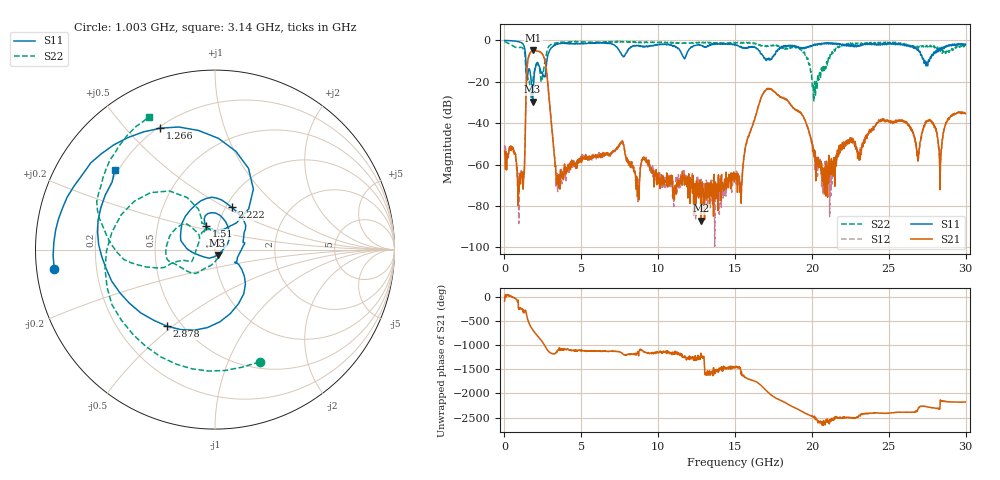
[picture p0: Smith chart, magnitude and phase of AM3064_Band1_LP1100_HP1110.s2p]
# Hz S DB R 50.0
!freq dBS11 angS11 dBS21 angS21 dBS12 angS12 dBS22 angS22
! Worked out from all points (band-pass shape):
!   1600 points, 10 MHz to 29.98 GHz, reference 50 ohm
!   highest |S21| = -4.83 dB at 1.884 GHz (marker M1); lowest = -87.1 dB at 12.77 GHz (marker M2)
!   |S21| within 3 dB of the highest: 1.578 GHz to 2.553 GHz (975.3 MHz wide, 47.2 % of centre)
!   lowest |S11| = -29.7 dB at 1.828 GHz (marker M3), VSWR 1.07, Z = 51.4 - j3.04 ohm
!   |S11| at or under -10 dB: 1.393 GHz to 2.759 GHz (1.366 GHz wide, 65.8 % of centre); 27.28266 GHz to 27.35234 GHz (69.67 MHz wide, 0.255 % of centre); 27.36 GHz to 27.57 GHz (208.9 MHz wide, 0.761 % of centre)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
!   |S22| runs from -29.5 to -0.5 dB; largest |S21 - S12| = 0.008
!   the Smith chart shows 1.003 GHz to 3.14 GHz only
!   S11 on the Smith chart (normalised r, x): 1.003 GHz: 0.05, -0.06; 1.266 GHz: 0.21, +0.63; 1.51 GHz: 0.88, +0.24; 2.222 GHz: 1.06, +0.54; 2.878 GHz: 0.42, -0.48; 3.14 GHz: 0.19, +0.34
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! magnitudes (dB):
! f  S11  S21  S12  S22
! 10 MHz  -0.1  -53.6  -50.6  -0.5
! 1.003 GHz  -0.9  -65.0  -65.7  -3.4
! 1.266 GHz  -2.6  -63.7  -65.3  -4.7
! 1.51 GHz  -17.1  -10.3  -10.3  -18.9
! 1.828 GHz  -29.7  -4.9  -5.0  -20.3
! 1.884 GHz  -22.7  -4.8  -4.9  -17.4
! 2.222 GHz  -11.9  -5.3  -5.3  -12.5
! 2.878 GHz  -6.0  -25.7  -25.7  -3.0
! 3.14 GHz  -2.9  -47.1  -46.9  -1.7
! 3.478 GHz  -1.8  -67.5  -72.2  -1.1
! 5.015 GHz  -1.4  -58.9  -57.1  -0.6
! 7.62 GHz  -7.0  -49.3  -48.9  -0.7
! 8.651 GHz  -2.6  -75.5  -69.7  -0.8
! 10 GHz  -2.1  -67.9  -63.6  -0.9
! 12.77 GHz  -2.4  -87.1  -71.5  -1.1
! 15 GHz  -2.2  -64.6  -66.7  -1.4
! 17.1 GHz  -9.1  -23.4  -23.4  -2.6
! 19.99 GHz  -3.0  -49.1  -49.3  -17.9
! 21.1 GHz  -1.5  -55.5  -69.1  -8.7
! 25 GHz  -1.3  -39.0  -38.7  -1.2
! 28.35 GHz  -4.8  -61.2  -66.2  -5.3
! 29.98 GHz  -1.8  -35.4  -34.9  -2.9
